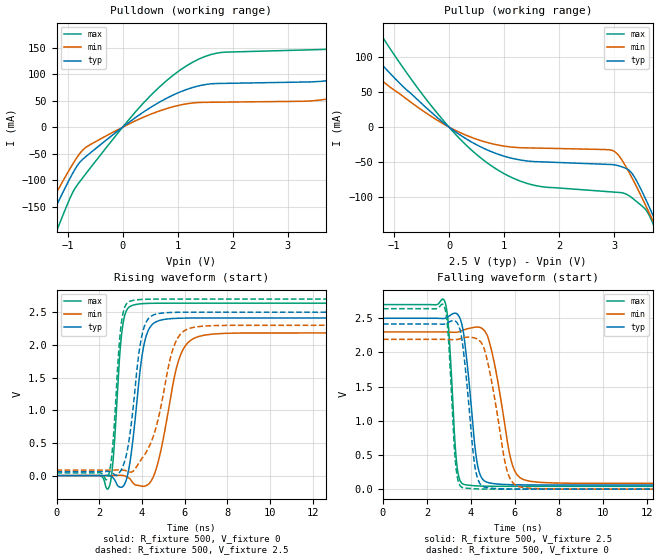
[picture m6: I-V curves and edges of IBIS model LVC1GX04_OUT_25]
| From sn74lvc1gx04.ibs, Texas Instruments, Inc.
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[Model]   LVC1GX04_OUT_25
Model_type  Output
Vref =   0
Rref =   500
Cref =   30p
Vmeas =   1.25
| variable   typ   min   max
C_comp   9.80pF   6.16pF   14.74pF
| C_pullup   9.65pF   6.16pF   11.31pF
| C_pulldown   9.96pF   6.68pF   14.74pF
[Temperature Range]   40   100   -40
| Ambient temperature   25   85   -40
[Voltage range]   2.5   2.3   2.7
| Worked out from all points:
|   slope of the pulldown table from 0 to 0.375 V, typ, clamps not added: 13.3 ohm
|   slope of the pullup table from 0 to 0.375 V, typ, clamps not added: 19 ohm
|   rising waveform, R_fixture 500, V_fixture 0: 20-80 % time 501ps typ, 784ps min, 315ps max; typ from 0 V to 2.41 V
|   falling waveform, R_fixture 500, V_fixture 2.5: 20-80 % time 442ps typ, 696ps min, 276ps max; typ from 2.5 V to 0.061 V
|   rising waveform, R_fixture 500, V_fixture 2.5: 20-80 % time 524ps typ, 933ps min, 321ps max; typ from 0.061 V to 2.5 V
|   falling waveform, R_fixture 500, V_fixture 0: 20-80 % time 428ps typ, 693ps min, 266ps max; typ from 2.42 V to 0 V
[Pulldown]
| LVC1GX04_OUT_25
|   Voltage   I(typ)   I(min)   I(max)
-5.5V     -1.06A     -941.4mA   -1.275A
-1.52V    -217.1mA   -184.1mA   -281.2mA
-1.26V    -160.6mA   -134.6mA   -212.3mA
-665mV    -55.38mA   -37.96mA   -87.52mA
385mV     28.96mA    19.04mA    46.35mA
1.275V    74.94mA    45.66mA    122.7mA
3.82V     89.63mA    55.12mA    148.2mA
5.34V     157.4mA    105.8mA    232mA
5.91V     188.7mA    52.55mA    283.4mA
6.525V    93.54mA    53.06mA    299.5mA
7.555V    94.08mA    54.03mA    161.4mA
11V       99.63mA    57.49mA    169.6mA
[Pullup]
| LVC1GX04_OUT_25
|   Voltage   I(typ)   I(min)   I(max)
-5.5V     533.4mA    418.6mA    746.4mA
-2.335V   192.2mA    147mA      274.9mA
-1.875V   147.9mA    112.2mA    212.9mA
-1.315V   97.38mA    72.9mA     141.5mA
-225mV    14.47mA    10.42mA    20.98mA
735mV     -33.88mA   -22.76mA   -53.28mA
1.56V     -49.18mA   -29.79mA   -83.17mA
2.98V     -53.48mA   -33.7mA    -92.52mA
3.325V    -66.27mA   -72.72mA   -100.9mA
3.755V    -135mA     -142.5mA   -147.1mA
3.835V    -149.5mA   -156.2mA   -162.8mA
11V       -1.609A    -1.492A    -1.841A
[Ramp]
| LVC1GX04_OUT_25
| variable   typ   min   max
dV/dt_r   1.55/5.41E-10   1.41/8.45E-10   1.71/3.47E-10
dV/dt_f   1.51/4.62E-10   1.37/7.25E-10   1.64/2.97E-10
R_load = 500
[Rising Waveform]
| LVC1GX04_OUT_25
R_fixture =   500
C_fixture =   0
L_fixture =   0
V_fixture =   0
V_fixture_min = 0
V_fixture_max = 0
|   Time   V(typ)   V(min)   V(max)
0s        125.3pV    6.247nV    2.314nV
2.46ns    2.227mV    -65.47uV   -178.4mV
2.66ns    -37.01mV   745.9uV    270.2mV
3.085ns   -172.9mV   3.344mV    2.252V
3.585ns   559.3mV    -112.7mV   2.607V
3.99ns    1.793V     -160.8mV   2.629V
4.325ns   2.237V     -126.7mV   2.634V
5.74ns    2.407V     1.78V      2.637V
6.625ns   2.41V      2.124V     2.637V
24.99ns   2.411V     2.183V     2.637V
[Falling Waveform]
| LVC1GX04_OUT_25
R_fixture =   500
C_fixture =   0
L_fixture =   0
V_fixture =   2.5
V_fixture_min = 2.3
V_fixture_max = 2.7
|   Time   V(typ)   V(min)   V(max)
0s        2.5V       2.3V       2.7V
2.8ns     2.497V     2.3V       2.756V
2.985ns   2.526V     2.298V     2.37V
3.36ns    2.567V     2.296V     367.3mV
3.695ns   2.223V     2.331V     68.62mV
4.275ns   408.6mV    2.372V     48.02mV
4.775ns   97.71mV    2.227V     43.45mV
5.83ns    65.57mV    424.5mV    41.71mV
6.44ns    62.63mV    135mV      41.58mV
24.99ns   60.95mV    83.67mV    41.48mV
[Rising Waveform]
| LVC1GX04_OUT_25
R_fixture =   500
C_fixture =   0
L_fixture =   0
V_fixture =   2.5
V_fixture_min = 2.3
V_fixture_max = 2.7
|   Time   V(typ)   V(min)   V(max)
0s        60.91mV    83.6mV     41.45mV
2.4ns     65.04mV    83.52mV    -28.72mV
2.62ns    40.4mV     84.04mV    404.5mV
3.035ns   88.65mV    87.99mV    2.32V
3.485ns   741.9mV    54.29mV    2.672V
3.885ns   1.925V     204.8mV    2.692V
4.2ns     2.348V     357.7mV    2.697V
5.485ns   2.496V     1.961V     2.7V
6.23ns    2.499V     2.252V     2.7V
24.99ns   2.5V       2.3V       2.7V
[Falling Waveform]
| LVC1GX04_OUT_25
R_fixture =   500
C_fixture =   0
L_fixture =   0
V_fixture =   0
V_fixture_min = 0
V_fixture_max = 0
|   Time   V(typ)   V(min)   V(max)
0s        2.416V     2.191V     2.64V
2.78ns    2.413V     2.191V     2.683V
2.97ns    2.438V     2.19V      2.259V
3.31ns    2.456V     2.188V     363mV
3.615ns   2.146V     2.211V     23.2mV
4.18ns    345.8mV    2.211V     5.736mV
4.625ns   30.81mV    2.037V     1.909mV
5.61ns    3.553mV    318.5mV    269.5uV
6.2ns     1.243mV    35.84mV    129.1uV
24.99ns   42.66uV    64.02uV    29.19uV
